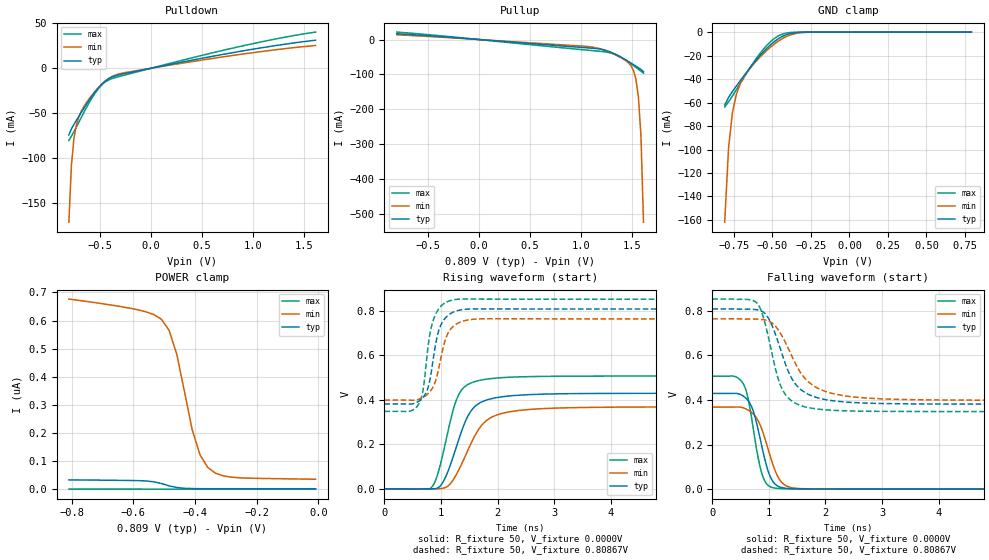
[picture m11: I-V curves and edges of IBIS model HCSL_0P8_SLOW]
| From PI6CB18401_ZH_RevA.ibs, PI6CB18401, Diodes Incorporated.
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[Model]   HCSL_0P8_SLOW
Model_type Output
Vref=0.8000V
Vmeas=900mV
| variable   typ   min   max
C_comp   2.000pF   1.970pF   2.030pF
[Voltage Range]   0.80867V   0.76428V   0.85294V
[POWER Clamp Reference]   0.80867V   0.76428V   0.85294V
[GND Clamp Reference]   0.0000V   0.0000V   0.0000V
[Pullup Reference]   0.80867V   0.76428V   0.85294V
[Pulldown Reference]   0.0000V   0.0000V   0.0000V
[Temperature Range]   25   85   -40
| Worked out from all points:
|   slope of the pulldown table from 0 to 0.121 V, typ, clamps not added: 43.9 ohm
|   slope of the pullup table from 0 to 0.121 V, typ, clamps not added: 43.9 ohm
|   GND clamp passes 1 mA (typ) near -0.37 V on its own axis
|   falling waveform, R_fixture 50, V_fixture 0.0000V: 20-80 % time 248ps typ, 292ps min, 210ps max; typ from 0.43 V to 0 V
|   rising waveform, R_fixture 50, V_fixture 0.0000V: 20-80 % time 379ps typ, 459ps min, 300ps max; typ from 0 V to 0.43 V
|   falling waveform, R_fixture 50, V_fixture 0.80867V: 20-80 % time 412ps typ, 523ps min, 311ps max; typ from 0.809 V to 0.382 V
|   rising waveform, R_fixture 50, V_fixture 0.80867V: 20-80 % time 194ps typ, 224ps min, 170ps max; typ from 0.382 V to 0.809 V
[GND Clamp]
| Voltage   I(typ)   I(min)   I(max)
-808.7mV  -62.12mA   -161.9mA   -63.86mA
-783.7mV  -55.6mA    -98.8mA    -59.36mA
-758.7mV  -50.64mA   -68.72mA   -54.46mA
-733.7mV  -46.08mA   -53.26mA   -49.26mA
-708.7mV  -41.61mA   -44.26mA   -43.9mA
-658.7mV  -32.83mA   -33.35mA   -33.29mA
-558.7mV  -16.95mA   -18.51mA   -14.73mA
-483.7mV  -7.773mA   -9.828mA   -5.14mA
-408.7mV  -2.206mA   -3.768mA   -815.3uA
-358.7mV  -647.7uA   -1.514mA   -143.2uA
-283.7mV  -64.34uA   -253.4uA   -5.991uA
791.3mV   1.208nA    35.61nA    1.246pA
[POWER Clamp]
| Voltage   I(typ)   I(min)   I(max)
-808.7mV  33.02nA    676.5nA    257.7pA
-583.7mV  30.32nA    637.8nA    188.8pA
-533.7mV  26.33nA    621.5nA    64.6pA
-508.7mV  20.08nA    604.6nA    40.81pA
-483.7mV  11.74nA    565.4nA    32.71pA
-458.7mV  5.847nA    479.8nA    29.42pA
-408.7mV  2.125nA    211.3nA    26.04pA
-383.7mV  1.712nA    122.8nA    24.68pA
-358.7mV  1.545nA    77.92nA    23.35pA
-333.7mV  1.471nA    57.06nA    22.03pA
-258.7mV  1.389nA    40.71nA    18.09pA
-8.67mV   1.225nA    35.32nA    4.944pA
[Pulldown]
| Voltage   I(typ)   I(min)   I(max)
-808.7mV  -74.27mA   -171.4mA   -80.33mA
-783.7mV  -67.64mA   -108.2mA   -75.67mA
-758.7mV  -62.54mA   -78.03mA   -70.61mA
-733.7mV  -57.85mA   -62.46mA   -65.22mA
-683.7mV  -48.67mA   -47.13mA   -54.12mA
-633.7mV  -39.76mA   -37.93mA   -43.34mA
-533.7mV  -23.94mA   -23.52mA   -25.04mA
-433.7mV  -12.87mA   -12.77mA   -14.02mA
-308.7mV  -7.139mA   -6.169mA   -9.062mA
116.3mV   2.651mA    2.176mA    3.424mA
966.3mV   20.53mA    16.79mA    26.52mA
1.616V    31.19mA    25.32mA    40.23mA
[Pullup]
| Voltage   I(typ)   I(min)   I(max)
-808.7mV  16.57mA    13.58mA    21.32mA
1.091V    -24.38mA   -20.82mA   -31.08mA
1.191V    -27.61mA   -26.52mA   -33.84mA
1.291V    -35.78mA   -37.17mA   -38.25mA
1.366V    -45.82mA   -47.55mA   -46.33mA
1.441V    -58.07mA   -60.28mA   -58.88mA
1.491V    -66.98mA   -74.13mA   -68.92mA
1.516V    -71.53mA   -87.43mA   -74.27mA
1.541V    -76.11mA   -112.5mA   -79.76mA
1.566V    -80.77mA   -164.2mA   -85.31mA
1.591V    -85.8mA    -275.9mA   -90.8mA
1.616V    -92.3mA    -522.6mA   -96.1mA
[Falling Waveform]
R_fixture = 50
V_fixture = 0.0000V
V_fixture_min = 0.0000V
V_fixture_max = 0.0000V
|   Time   V(typ)   V(min)   V(max)
0s        429.6mV    368.3mV    507.1mV
390ps     430mV      368.4mV    506.3mV
555ps     416mV      364.1mV    468.9mV
630ps     398.1mV    355.4mV    409.7mV
705ps     363.3mV    341.9mV    301.7mV
855ps     215.3mV    282.2mV    89.35mV
1.035ns   50.19mV    138.5mV    9.534mV
1.2ns     9.145mV    39.02mV    2.691mV
1.44ns    2.149mV    5.076mV    1.271mV
5ns       27.78uV    38.38uV    22.46uV
[Rising Waveform]
R_fixture = 50
V_fixture = 0.0000V
V_fixture_min = 0.0000V
V_fixture_max = 0.0000V
|   Time   V(typ)   V(min)   V(max)
0s        10.48uV    11.11uV    10.51uV
840ps     -114.9uV   -136.3uV   8.275mV
940ps     3.402mV    328.8uV    63.74mV
1.04ns    32.09mV    2.651mV    163.1mV
1.3ns     210.3mV    77.45mV    416.5mV
1.5ns     338mV      186.9mV    472.4mV
1.7ns     388mV      279.3mV    488.6mV
2.08ns    413.8mV    339mV      499.9mV
2.9ns     426.3mV    361.7mV    505.8mV
10ns      429.6mV    368.3mV    507.1mV
[Falling Waveform]
R_fixture = 50
V_fixture = 0.80867V
V_fixture_min = 0.76428V
V_fixture_max = 0.85294V
|   Time   V(typ)   V(min)   V(max)
0s        808.7mV    764.3mV    852.9mV
800ps     804.4mV    762.8mV    831.8mV
1ns       763mV      754.1mV    672.4mV
1.14ns    677.6mV    723.9mV    516.3mV
1.24ns    601.2mV    683.6mV    446.3mV
1.44ns    482mV      578.9mV    389.8mV
1.68ns    427.7mV    486.1mV    367mV
2.15ns    396.1mV    427.9mV    353.7mV
3ns       384.4mV    405.2mV    349.1mV
10ns      381.5mV    398.7mV    348.2mV
[Rising Waveform]
R_fixture = 50
V_fixture = 0.80867V
V_fixture_min = 0.76428V
V_fixture_max = 0.85294V
|   Time   V(typ)   V(min)   V(max)
0s        381.5mV    398.7mV    348.2mV
445ps     380.9mV    398.7mV    348.9mV
610ps     394.4mV    403.1mV    382.6mV
685ps     412mV      411.6mV    446.6mV
760ps     447.1mV    425.2mV    615mV
850ps     561mV      453.8mV    746.7mV
955ps     707mV      536mV      807.4mV
1.135ns   782.2mV    705.1mV    843.9mV
1.65ns    809.3mV    763.9mV    853.3mV
5ns       808.7mV    764.3mV    852.9mV
[Ramp]
| variable   typ   min   max
dV/dt_r   0.25777V/378.83p   0.22106V/459.48p   0.30431V/300.24p
dV/dt_f   0.25619V/412.14p   0.21911V/521.99p   0.30283V/310.79p
R_load = 50
